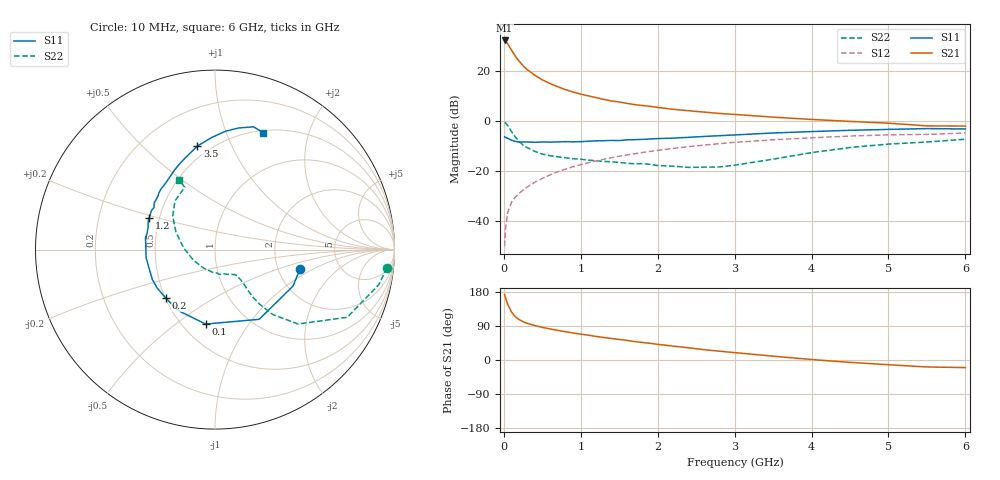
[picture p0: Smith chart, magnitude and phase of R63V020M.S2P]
! SIEMENS Small Signal Semiconductors
! BFR193
! Si NPN RF Bipolar Junction Transistor in SOT23
! VCE = 3 V  IC = 20 mA
! Common Emitter S-Parameters:  May  1996
# GHz  S  MA  R  50
!  f  S11  S21  S12  S22
! GHz  MAG  ANG  MAG  ANG  MAG  ANG  MAG  ANG
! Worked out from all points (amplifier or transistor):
!   36 points, 10 MHz to 6 GHz, reference 50 ohm
!   highest |S21| = 32.3 dB at 10 MHz (marker M1)
!   |S21| within 3 dB of that: start of sweep to 83.06 MHz
!   unconditionally stable (mu >= 1): 552.3 MHz to 1.849 GHz
!   at 250 MHz: K = 0.83, MSG = 24.8 dB, |S12| = -27.4 dB
!   at 1.4 GHz: K = 1.03, MAG = 10.3 dB, |S12| = -14.5 dB
!   at 6 GHz: K = 0.95, MSG = 1.4 dB, |S12| = -4.6 dB
!   lowest NFmin = 1.40 dB at 450 MHz
!   S11 on the Smith chart (normalised r, x): 10 MHz: 2.65, -0.75; 100 MHz: 0.65, -0.65; 200 MHz: 0.50, -0.32; 1.2 GHz: 0.44, +0.18; 3.5 GHz: 0.43, +0.75; 6 GHz: 0.53, +1.36
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0.01  0.4869 -12.8  41.39 172.6  0.0032 85.1  0.9627 -6.0
0.02  0.4794 -25.2  40.46 165.3  0.0066 80.8  0.9341 -12.0
0.05  0.4599 -57.6  35.66 146.9  0.0151 70.6  0.8279 -27.1
0.1  0.4181 -97.1  26.5 126.3  0.0242 63.1  0.6206 -41.9
0.15  0.3966 -121.0  19.93 114.1  0.0308 62.1  0.485 -48.3
0.2  0.3851 -135.4  15.85 106.5  0.0364 63.2  0.3957 -50.7
0.25  0.3868 -146.6  12.94 100.9  0.0425 64.6  0.3361 -51.5
0.3  0.3868 -154.4  10.94 97.0  0.0483 66.0  0.3008 -51.2
0.4  0.3818 -165.2  8.416 91.1  0.0604 67.3  0.2526 -50.1
0.5  0.3865 -173.1  6.76 86.0  0.0722 68.5  0.2223 -49.6
0.6  0.385 -179.7  5.707 82.0  0.085 68.9  0.2065 -49.8
0.8  0.3929 170.7  4.303 74.6  0.1107 68.2  0.1874 -50.3
1  0.3929 161.5  3.492 68.3  0.1363 67.0  0.1747 -52.8
1.1  0.4004 158.6  3.226 65.4  0.1495 66.2  0.1677 -55.3
1.2  0.4077 154.7  2.982 62.2  0.1622 65.1  0.1629 -57.4
1.4  0.4156 148.2  2.556 56.8  0.1875 63.0  0.1559 -62.2
1.7  0.431 139.3  2.161 48.5  0.2252 59.3  0.1419 -71.8
2.2  0.4617 126.4  1.743 36.6  0.2875 52.7  0.1273 -96.4
3.5  0.5855 99.6  1.214 10.1  0.4277 33.0  0.1754 176.5
4.5  0.6624 84.9  0.998 -6.3  0.5082 18.6  0.3002 141.7
5.5  0.7168 72.6  0.812 -18.4  0.5484 4.3  0.3862 115.9
6  0.7048 67.5  0.805 -20.0  0.5855 0.1  0.4395 117.3
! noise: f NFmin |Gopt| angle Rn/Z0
0.45  1.4  0.3  160  0.1
0.9  1.45  0.34  172  0.11
1.8  2.2  0.56  -148  0.2
